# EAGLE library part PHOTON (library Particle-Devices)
Particle Photon Wi-Fi through-hole development board footprint Product datasheet: here Design files: here Github : Particle devices library
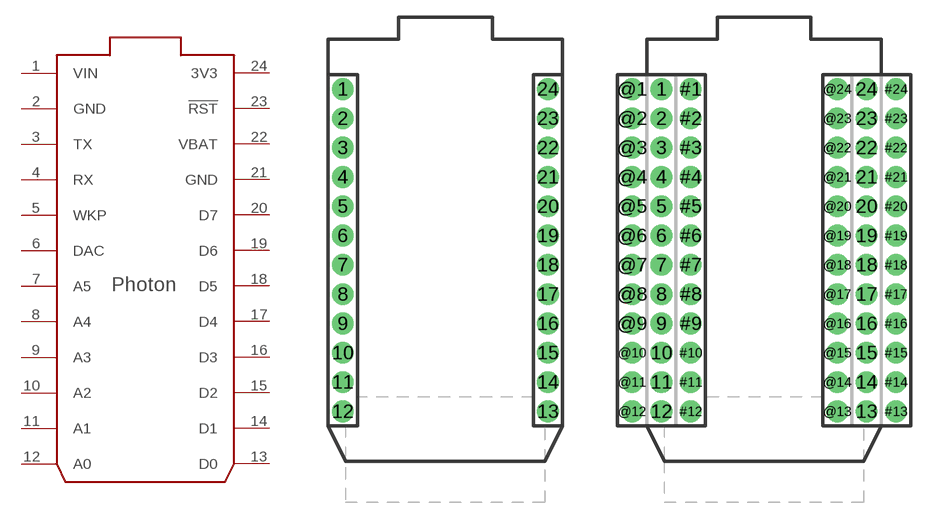
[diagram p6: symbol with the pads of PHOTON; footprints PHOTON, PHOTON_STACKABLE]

Designator prefix -

## PHOTON_WITH_HEADERS  [PHOTON]
1  VIN  pwr
2  GND  pwr
3  TX
4  RX
5  WKP
6  DAC
7  A5
8  A4
9  A3
10  A2
11  A1
12  A0
13  D0
14  D1
15  D2
16  D3
17  D4
18  D5
19  D6
20  D7
21  GND  pwr
22  VBAT  pwr
23  !RST
24  3V3  pwr

## PHOTON_WITH_STACKABLE_HEADERS  [PHOTON_STACKABLE]
1  VIN  pwr
2  GND  pwr
3  TX
4  RX
5  WKP
6  DAC
7  A5
8  A4
9  A3
10  A2
11  A1
12  A0
13  D0
14  D1
15  D2
16  D3
17  D4
18  D5
19  D6
20  D7
21  GND  pwr
22  VBAT  pwr
23  !RST
24  3V3  pwr
#1  VIN  pwr
#2  GND  pwr
#3  TX
#4  RX
#5  WKP
#6  DAC
#7  A5
#8  A4
#9  A3
#10  A2
#11  A1
#12  A0
#13  D0
#14  D1
#15  D2
#16  D3
#17  D4
#18  D5
#19  D6
#20  D7
#21  GND  pwr
#22  VBAT  pwr
#23  !RST
#24  3V3  pwr
@1  VIN  pwr
@2  GND  pwr
@3  TX
@4  RX
@5  WKP
@6  DAC
@7  A5
@8  A4
@9  A3
@10  A2
@11  A1
@12  A0
@13  D0
@14  D1
@15  D2
@16  D3
@17  D4
@18  D5
@19  D6
@20  D7
@21  GND  pwr
@22  VBAT  pwr
@23  !RST
@24  3V3  pwr

## Footprint PHOTON (pad centres in mm)
drill 1.016 pad 1.88: 1 1.27,33.02; 2 1.27,30.48; 3 1.27,27.94; 4 1.27,25.4; 5 1.27,22.86; 6 1.27,20.32; 7 1.27,17.78; 8 1.27,15.24; 9 1.27,12.7; 10 1.27,10.16; 11 1.27,7.62; 12 1.27,5.08; 13 19.05,5.08; 14 19.05,7.62; 15 19.05,10.16; 16 19.05,12.7; 17 19.05,15.24; 18 19.05,17.78; 19 19.05,20.32; 20 19.05,22.86; 21 19.05,25.4; 22 19.05,27.94; 23 19.05,30.48; 24 19.05,33.02

## Footprint PHOTON_STACKABLE (pad centres in mm)
drill 1.016 pad 1.88: 1 1.27,33.02; 2 1.27,30.48; 3 1.27,27.94; 4 1.27,25.4; 5 1.27,22.86; 6 1.27,20.32; 7 1.27,17.78; 8 1.27,15.24; 9 1.27,12.7; 10 1.27,10.16; 11 1.27,7.62; 12 1.27,5.08; 13 19.05,5.08; 14 19.05,7.62; 15 19.05,10.16; 16 19.05,12.7; 17 19.05,15.24; 18 19.05,17.78; 19 19.05,20.32; 20 19.05,22.86; 21 19.05,25.4; 22 19.05,27.94; 23 19.05,30.48; 24 19.05,33.02; #1 3.81,33.02; #2 3.81,30.48; #3 3.81,27.94; #4 3.81,25.4; #5 3.81,22.86; #6 3.81,20.32; #7 3.81,17.78; #8 3.81,15.24; #9 3.81,12.7; #10 3.81,10.16; #11 3.81,7.62; #12 3.81,5.08; #13 21.59,5.08; #14 21.59,7.62; #15 21.59,10.16; #16 21.59,12.7; #17 21.59,15.24; #18 21.59,17.78; #19 21.59,20.32; #20 21.59,22.86; #21 21.59,25.4; #22 21.59,27.94; #23 21.59,30.48; #24 21.59,33.02; @1 -1.27,33.02; @2 -1.27,30.48; @3 -1.27,27.94; @4 -1.27,25.4; @5 -1.27,22.86; @6 -1.27,20.32; @7 -1.27,17.78; @8 -1.27,15.24; @9 -1.27,12.7; @10 -1.27,10.16; @11 -1.27,7.62; @12 -1.27,5.08; @13 16.51,5.08; @14 16.51,7.62; @15 16.51,10.16; @16 16.51,12.7; @17 16.51,15.24; @18 16.51,17.78; @19 16.51,20.32; @20 16.51,22.86; @21 16.51,25.4; @22 16.51,27.94; @23 16.51,30.48; @24 16.51,33.02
